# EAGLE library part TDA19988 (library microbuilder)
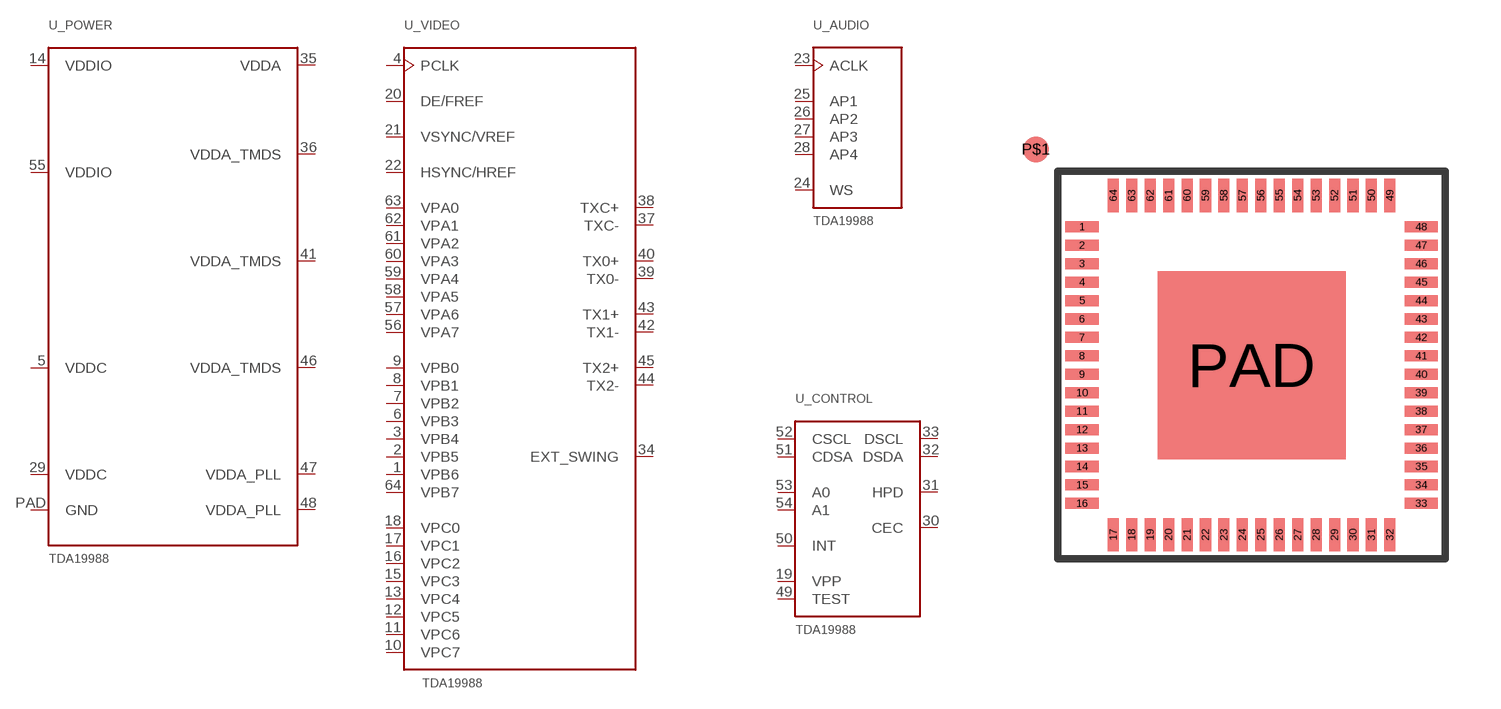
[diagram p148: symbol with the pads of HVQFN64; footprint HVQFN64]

Designator prefix U; gates _AUDIO=TDA19988_AUDIO _CONTROL=TDA19988_CTRL _POWER=TDA19988_PWR _VIDEO=TDA19988_VIDEO

## TDA19988  [HVQFN64]
1  _VIDEO:VPB6  in
2  _VIDEO:VPB5  in
3  _VIDEO:VPB4  in
4  _VIDEO:PCLK  in
5  _POWER:VDDC  pwr
6  _VIDEO:VPB3  in
7  _VIDEO:VPB2  in
8  _VIDEO:VPB1  in
9  _VIDEO:VPB0  in
10  _VIDEO:VPC7  in
11  _VIDEO:VPC6  in
12  _VIDEO:VPC5  in
13  _VIDEO:VPC4  in
14  _POWER:VDDIO  pwr
15  _VIDEO:VPC3  in
16  _VIDEO:VPC2  in
17  _VIDEO:VPC1  in
18  _VIDEO:VPC0  in
19  _CONTROL:VPP
20  _VIDEO:DE/FREF  in
21  _VIDEO:VSYNC/VREF  in
22  _VIDEO:HSYNC/HREF  in
23  _AUDIO:ACLK  in
24  _AUDIO:WS  in
25  _AUDIO:AP1  in
26  _AUDIO:AP2  in
27  _AUDIO:AP3  in
28  _AUDIO:AP4  in
29  _POWER:VDDC  pwr
30  _CONTROL:CEC
31  _CONTROL:HPD
32  _CONTROL:DSDA
33  _CONTROL:DSCL
34  _VIDEO:EXT_SWING  out
35  _POWER:VDDA  pwr
36  _POWER:VDDA_TMDS  pwr
37  _VIDEO:TXC-  out
38  _VIDEO:TXC+  out
39  _VIDEO:TX0-  out
40  _VIDEO:TX0+  out
41  _POWER:VDDA_TMDS  pwr
42  _VIDEO:TX1-  out
43  _VIDEO:TX1+  out
44  _VIDEO:TX2-  out
45  _VIDEO:TX2+  out
46  _POWER:VDDA_TMDS  pwr
47  _POWER:VDDA_PLL  pwr
48  _POWER:VDDA_PLL  pwr
49  _CONTROL:TEST
50  _CONTROL:INT
51  _CONTROL:CDSA
52  _CONTROL:CSCL
53  _CONTROL:A0
54  _CONTROL:A1
55  _POWER:VDDIO  pwr
56  _VIDEO:VPA7  in
57  _VIDEO:VPA6  in
58  _VIDEO:VPA5  in
59  _VIDEO:VPA4  in
60  _VIDEO:VPA3  in
61  _VIDEO:VPA2  in
62  _VIDEO:VPA1  in
63  _VIDEO:VPA0  in
64  _VIDEO:VPB7  in
PAD  _POWER:GND  pwr

## Footprint HVQFN64 (pad centres in mm)
smd 0.9 x 0.3: 1 -4.6,3.75; 2 -4.6,3.25; 3 -4.6,2.75; 4 -4.6,2.25; 5 -4.6,1.75; 6 -4.6,1.25; 7 -4.6,0.75; 8 -4.6,0.25; 9 -4.6,-0.25; 10 -4.6,-0.75; 11 -4.6,-1.25; 12 -4.6,-1.75; 13 -4.6,-2.25; 14 -4.6,-2.75; 15 -4.6,-3.25; 16 -4.6,-3.75; 33 4.6,-3.75; 34 4.6,-3.25; 35 4.6,-2.75; 36 4.6,-2.25; 37 4.6,-1.75; 38 4.6,-1.25; 39 4.6,-0.75; 40 4.6,-0.25; 41 4.6,0.25; 42 4.6,0.75; 43 4.6,1.25; 44 4.6,1.75; 45 4.6,2.25; 46 4.6,2.75; 47 4.6,3.25; 48 4.6,3.75
smd 0.3 x 0.9: 17 -3.75,-4.6; 18 -3.25,-4.6; 19 -2.75,-4.6; 20 -2.25,-4.6; 21 -1.75,-4.6; 22 -1.25,-4.6; 23 -0.75,-4.6; 24 -0.25,-4.6; 25 0.25,-4.6; 26 0.75,-4.6; 27 1.25,-4.6; 28 1.75,-4.6; 29 2.25,-4.6; 30 2.75,-4.6; 31 3.25,-4.6; 32 3.75,-4.6; 49 3.75,4.6; 50 3.25,4.6; 51 2.75,4.6; 52 2.25,4.6; 53 1.75,4.6; 54 1.25,4.6; 55 0.75,4.6; 56 0.25,4.6; 57 -0.25,4.6; 58 -0.75,4.6; 59 -1.25,4.6; 60 -1.75,4.6; 61 -2.25,4.6; 62 -2.75,4.6; 63 -3.25,4.6; 64 -3.75,4.6
smd 0.7 x 0.7: P$1 -5.85,5.85
smd 5.1 x 5.1: PAD 0,0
